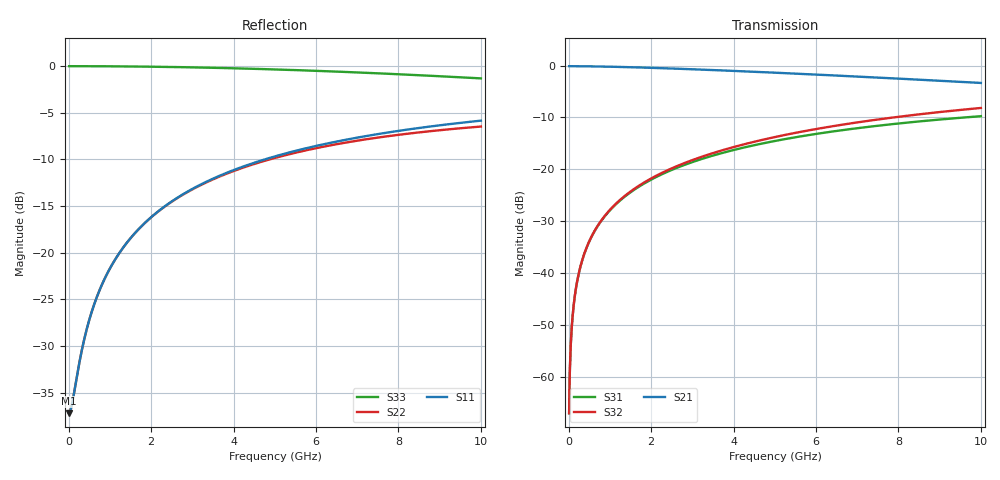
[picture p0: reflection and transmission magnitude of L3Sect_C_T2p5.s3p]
! Created Fri Sep 09 15:04:52 2011
# ghz S ma R 50
! 3 Port Network Data from SP1.SP block
! freq  magS11  angS11  magS12  angS12  magS13  angS13
!  magS21  angS21
!  magS22  angS22  magS23  angS23
!  magS31  angS31  magS32  angS32
!  magS33  angS33
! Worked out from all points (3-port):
!   1000 points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, 10 MHz to 10 GHz, reference 50 ohm
!   strongest paths, dB at 10 MHz, 2.51 GHz, 5.01 GHz, 7.51 GHz, 10 GHz:
!     S21: -0.1, -0.6, -1.4, -2.3, -3.4
!     S32: -67.1, -19.8, -13.8, -10.4, -8.2
!     S31: -67.1, -20.1, -14.5, -11.6, -9.8
!   lowest |S11| = -37.2 dB at 10 MHz (marker M1), VSWR 1.03, Z = 51.4 + j0.0825 ohm
!   |S11| at or under -10 dB: start of sweep to 4.754 GHz
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0.01  0.01379 3.3  0.9861 -0.1  0.000442 65.7
      0.9861 -0.1  0.01379 3.3  0.0004438 65.8
      0.000442 65.7  0.0004438 65.8  0.9996 -0.0
0.1  0.01627 29.5  0.9857 -0.7  0.004032 87.0
     0.9857 -0.7  0.01627 29.4  0.004053 87.2
     0.004032 87.0  0.004053 87.2  0.9996 -0.5
0.16  0.01938 41.4  0.9854 -1.1  0.006447 87.7
      0.9854 -1.1  0.01939 41.2  0.006482 88.0
      0.006447 87.7  0.006482 88.0  0.9996 -0.7
0.24  0.02449 51.6  0.9848 -1.7  0.009667 87.8
      0.9848 -1.7  0.0245 51.3  0.009721 88.4
      0.009667 87.8  0.009721 88.4  0.9995 -1.1
0.5  0.04374 64.9  0.9823 -3.5  0.02012 87.2
     0.9823 -3.5  0.04376 64.4  0.02026 88.3
     0.02012 87.2  0.02026 88.3  0.9992 -2.3
0.91  0.07547 69.0  0.976 -6.3  0.03652 85.6
      0.976 -6.3  0.07548 68.0  0.03691 87.5
      0.03652 85.6  0.03691 87.5  0.9983 -4.2
1.54  0.1226 68.0  0.9625 -10.5  0.06144 82.9
      0.9625 -10.5  0.1225 66.4  0.0626 86.0
      0.06144 82.9  0.0626 86.0  0.9958 -7.1
2.41  0.1826 64.2  0.9388 -15.9  0.09503 79.3
      0.9388 -15.9  0.182 61.6  0.09825 83.7
      0.09503 79.3  0.09825 83.7  0.9902 -11.1
5.01  0.3287 52.6  0.8529 -30.7  0.1875 69.0
      0.8529 -30.7  0.3225 47.4  0.2045 76.3
      0.1875 69.0  0.2045 76.3  0.9601 -22.9
10  0.5104 35.8  0.6795 -55.0  0.3247 52.8
    0.6795 -55.0  0.4745 27.0  0.3897 61.2
    0.3247 52.8  0.3897 61.2  0.8598 -44.3
